(* Logix 5000 AddOnInstructionDefinition export POINT_ENC; software revision 30.00; part 2 of 2 *)

ADD_ON_INSTRUCTION B256_CtoE   (* revision 1.0 20170916, vendor Kenneth A. Fischer *)
// Convert 256-bit value using 22 12-bit pieces into 256-bit value using 32 8-bit pieces
// Revision note:
// Rev1.0: 20170916 - Initial Release
VAR_IN_OUT
   Inp_C : DINT[22]; {required}
   Out_E : DINT[32]; {required}
END_VAR
VAR
   i : INT;
   j : INT;
   TEMP1 : DINT;
   TEMP2 : DINT;
   D_SHL : D_SHL;
   D_SHR : D_SHR;
END_VAR

ROUTINE Logic   (* ladder *)
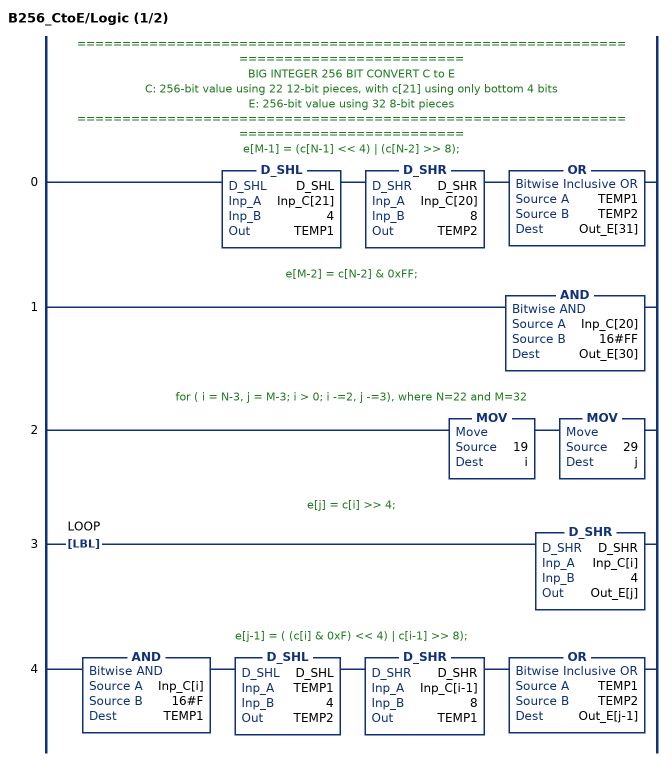
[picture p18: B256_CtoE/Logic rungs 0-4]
   // ======================================================================================
   // BIG INTEGER 256 BIT CONVERT C to E
   // C: 256-bit value using 22 12-bit pieces, with c[21] using only bottom 4 bits
   // E: 256-bit value using 32 8-bit pieces
   // ======================================================================================
   // e[M-1] = (c[N-1] << 4) | (c[N-2] >> 8);
   0: D_SHL(D_SHL,Inp_C[21],4,TEMP1)D_SHR(D_SHR,Inp_C[20],8,TEMP2)OR(TEMP1,TEMP2,Out_E[31]);
   // e[M-2] = c[N-2] & 0xFF;
   1: AND(Inp_C[20],16#FF,Out_E[30]);
   // for ( i = N-3, j = M-3; i > 0; i -=2, j -=3), where N=22 and M=32
   2: MOV(19,i)MOV(29,j);
   // e[j] = c[i] >> 4;
   3: LBL(LOOP)D_SHR(D_SHR,Inp_C[i],4,Out_E[j]);
   // e[j-1] = ( (c[i] & 0xF) << 4) | c[i-1] >> 8);
   4: AND(Inp_C[i],16#F,TEMP1)D_SHL(D_SHL,TEMP1,4,TEMP2)D_SHR(D_SHR,Inp_C[i-1],8,TEMP1)OR(TEMP1,TEMP2,Out_E[j-1]);
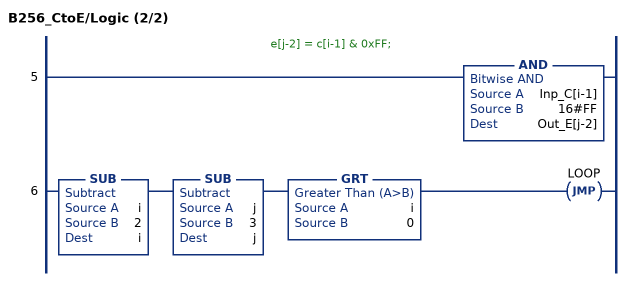
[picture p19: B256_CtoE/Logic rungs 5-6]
   // e[j-2] = c[i-1] & 0xFF;
   5: AND(Inp_C[i-1],16#FF,Out_E[j-2]);
   6: SUB(i,2,i)SUB(j,3,j)GRT(i,0)JMP(LOOP);
END_ROUTINE
END_ADD_ON_INSTRUCTION

ADD_ON_INSTRUCTION POINT_ENC   (* revision 1.0 20170916, vendor Kenneth A. Fischer *)
// Point Encode:
// Encode point (x,y) values into 32 8-bit pieces
// Requires POINT UDT
// Revision note:
// Rev1.0: 20170916 - Initial Release
VAR_IN_OUT
   Temp_C1 : DINT[22]; {required}
   Temp_C2 : DINT[22]; {required}
   Temp_C3 : DINT[22]; {required}
   Temp_C4 : DINT[22]; {required}   // U
   Temp_D : DINT[43]; {required}
   Temp_E : DINT[32]; {required}
   Inp_P : POINT; {required}
   Out_E : DINT[32]; {required}
END_VAR
VAR_OUTPUT
   i : INT; {access Read Only}
END_VAR
VAR_INPUT
   SEQCTRL_RESET : BOOL;   // Resets Point Multiplication if Toggled True
END_VAR
VAR_OUTPUT
   SEQCTRL_DN : BOOL; {access Read Only}   // Complete
   SEQCTRL_STEP : INT; {access Read Only}
END_VAR
VAR
   SEQCTRL_CMD : INT;
   SEQCTRL_DONE : INT;
   SEQCTRL_CMD_TABLE : INT[40];
   SEQCTRL_NEXT_STEP : INT;
   TEMP : INT;
   j : INT;
   b : DINT;
   B256_MUL : B256_MUL;
   B256_SQU : B256_SQU;
   B256_ADJ : B256_ADJ;
   B256_CtoE : B256_CtoE;
   D_SHL : D_SHL;
   TEMP1 : DINT;
   TEMP2 : DINT;
END_VAR

ROUTINE Logic   (* ladder *)
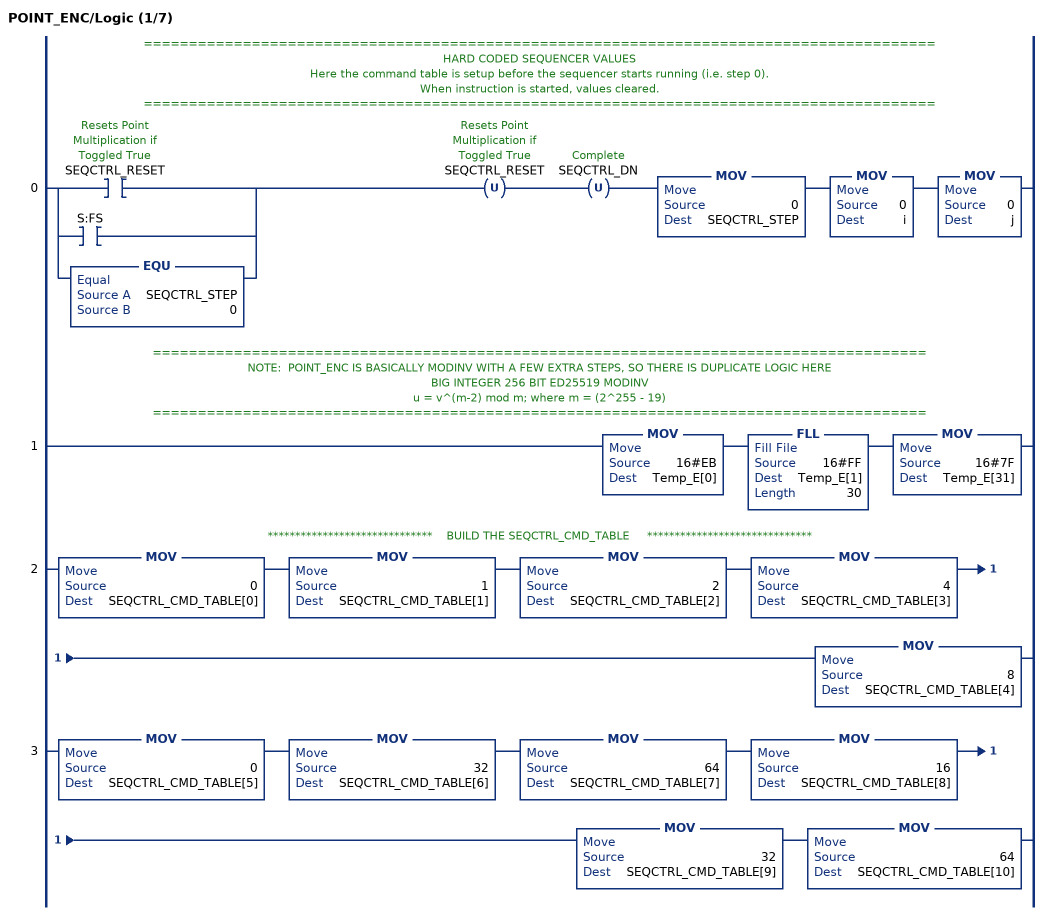
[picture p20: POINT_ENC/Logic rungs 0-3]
   // ========================================================================================
   // HARD CODED SEQUENCER VALUES
   // Here the command table is setup before the sequencer starts running (i.e. step 0).
   // When instruction is started, values cleared.
   // ========================================================================================
   0: [[XIC(SEQCTRL_RESET) ,XIC(S:FS) ] ,EQU(SEQCTRL_STEP,0) ]OTU(SEQCTRL_RESET)OTU(SEQCTRL_DN)MOV(0,SEQCTRL_STEP)MOV(0,i)MOV(0,j);
   // ======================================================================================
   // NOTE:  POINT_ENC IS BASICALLY MODINV WITH A FEW EXTRA STEPS, SO THERE IS DUPLICATE LOGIC HERE
   // BIG INTEGER 256 BIT ED25519 MODINV
   //  u = v^(m-2) mod m; where m = (2^255 - 19)
   // ======================================================================================
   1: MOV(16#EB,Temp_E[0])FLL(16#FF,Temp_E[1],30)MOV(16#7F,Temp_E[31]);
   // ******************************    BUILD THE SEQCTRL_CMD_TABLE     ******************************
   2: MOV(0,SEQCTRL_CMD_TABLE[0])MOV(1,SEQCTRL_CMD_TABLE[1])MOV(2,SEQCTRL_CMD_TABLE[2])MOV(4,SEQCTRL_CMD_TABLE[3])MOV(8,SEQCTRL_CMD_TABLE[4]);
   3: MOV(0,SEQCTRL_CMD_TABLE[5])MOV(32,SEQCTRL_CMD_TABLE[6])MOV(64,SEQCTRL_CMD_TABLE[7])MOV(16,SEQCTRL_CMD_TABLE[8])MOV(32,SEQCTRL_CMD_TABLE[9])MOV(64,SEQCTRL_CMD_TABLE[10]);
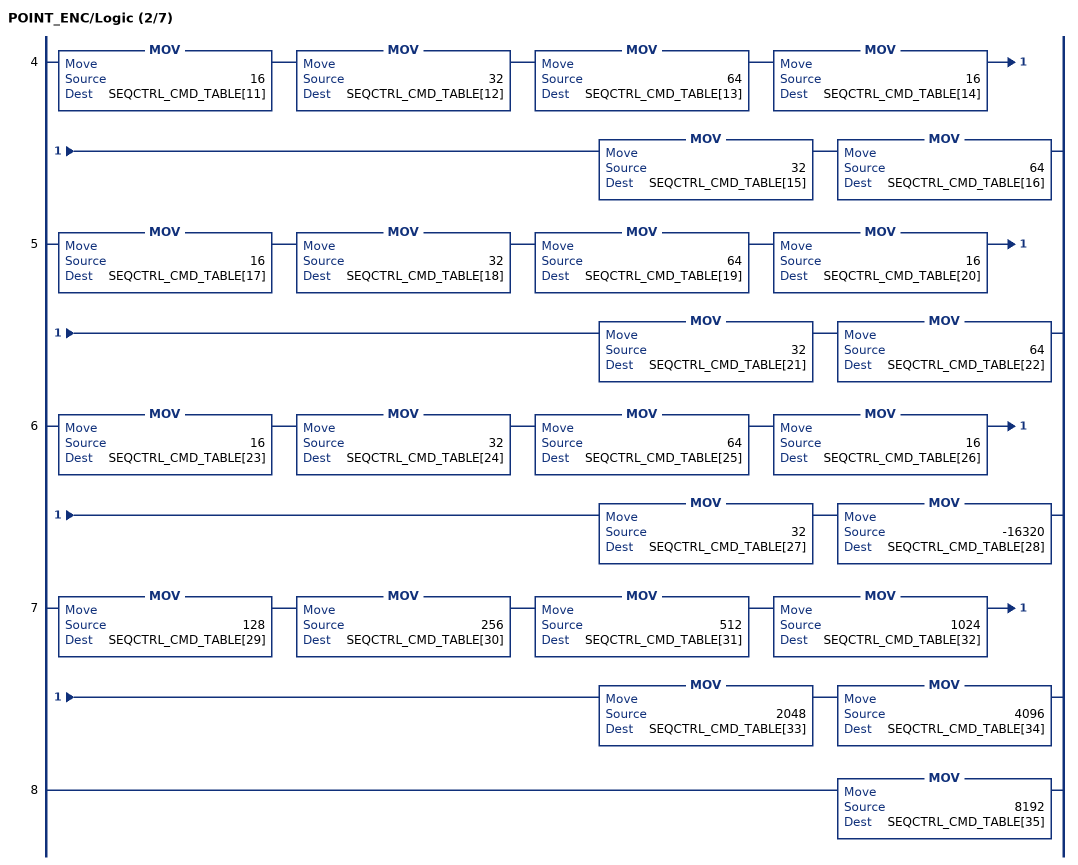
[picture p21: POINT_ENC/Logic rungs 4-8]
   4: MOV(16,SEQCTRL_CMD_TABLE[11])MOV(32,SEQCTRL_CMD_TABLE[12])MOV(64,SEQCTRL_CMD_TABLE[13])MOV(16,SEQCTRL_CMD_TABLE[14])MOV(32,SEQCTRL_CMD_TABLE[15])MOV(64,SEQCTRL_CMD_TABLE[16]);
   5: MOV(16,SEQCTRL_CMD_TABLE[17])MOV(32,SEQCTRL_CMD_TABLE[18])MOV(64,SEQCTRL_CMD_TABLE[19])MOV(16,SEQCTRL_CMD_TABLE[20])MOV(32,SEQCTRL_CMD_TABLE[21])MOV(64,SEQCTRL_CMD_TABLE[22]);
   6: MOV(16,SEQCTRL_CMD_TABLE[23])MOV(32,SEQCTRL_CMD_TABLE[24])MOV(64,SEQCTRL_CMD_TABLE[25])MOV(16,SEQCTRL_CMD_TABLE[26])MOV(32,SEQCTRL_CMD_TABLE[27])MOV(-16320,SEQCTRL_CMD_TABLE[28]);
   7: MOV(128,SEQCTRL_CMD_TABLE[29])MOV(256,SEQCTRL_CMD_TABLE[30])MOV(512,SEQCTRL_CMD_TABLE[31])MOV(1024,SEQCTRL_CMD_TABLE[32])MOV(2048,SEQCTRL_CMD_TABLE[33])MOV(4096,SEQCTRL_CMD_TABLE[34]);
   8: MOV(8192,SEQCTRL_CMD_TABLE[35]);
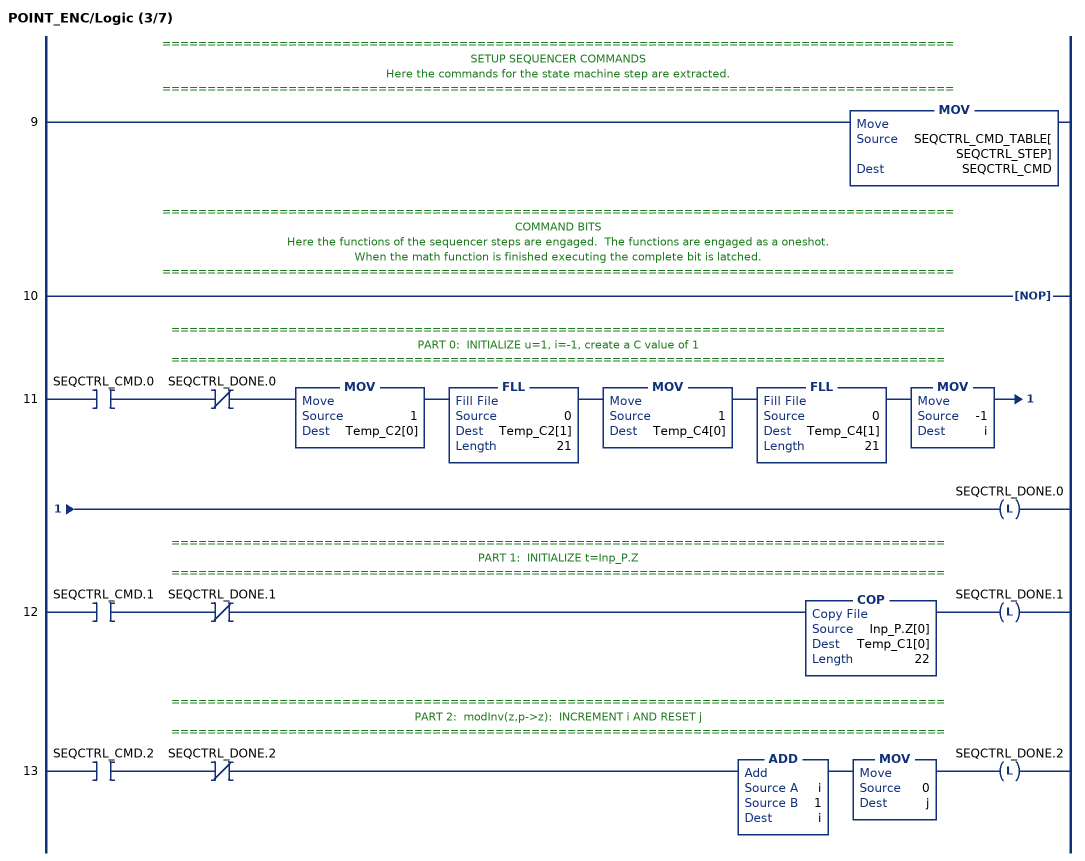
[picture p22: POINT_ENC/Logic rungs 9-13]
   // ========================================================================================
   // SETUP SEQUENCER COMMANDS
   // Here the commands for the state machine step are extracted.
   // ========================================================================================
   9: MOV(SEQCTRL_CMD_TABLE[SEQCTRL_STEP],SEQCTRL_CMD);
   // ========================================================================================
   // COMMAND BITS
   // Here the functions of the sequencer steps are engaged.  The functions are engaged as a oneshot.
   // When the math function is finished executing the complete bit is latched.
   // ========================================================================================
   10: NOP();
   // ======================================================================================
   // PART 0:  INITIALIZE u=1, i=-1, create a C value of 1
   // ======================================================================================
   11: XIC(SEQCTRL_CMD.0)XIO(SEQCTRL_DONE.0)MOV(1,Temp_C2[0])FLL(0,Temp_C2[1],21)MOV(1,Temp_C4[0])FLL(0,Temp_C4[1],21)MOV(-1,i)OTL(SEQCTRL_DONE.0);
   // ======================================================================================
   // PART 1:  INITIALIZE t=Inp_P.Z
   // ======================================================================================
   12: XIC(SEQCTRL_CMD.1)XIO(SEQCTRL_DONE.1)COP(Inp_P.Z[0],Temp_C1[0],22)OTL(SEQCTRL_DONE.1);
   // ======================================================================================
   // PART 2:  modInv(z,p->z):  INCREMENT i AND RESET j
   // ======================================================================================
   13: XIC(SEQCTRL_CMD.2)XIO(SEQCTRL_DONE.2)ADD(i,1,i)MOV(0,j)OTL(SEQCTRL_DONE.2);
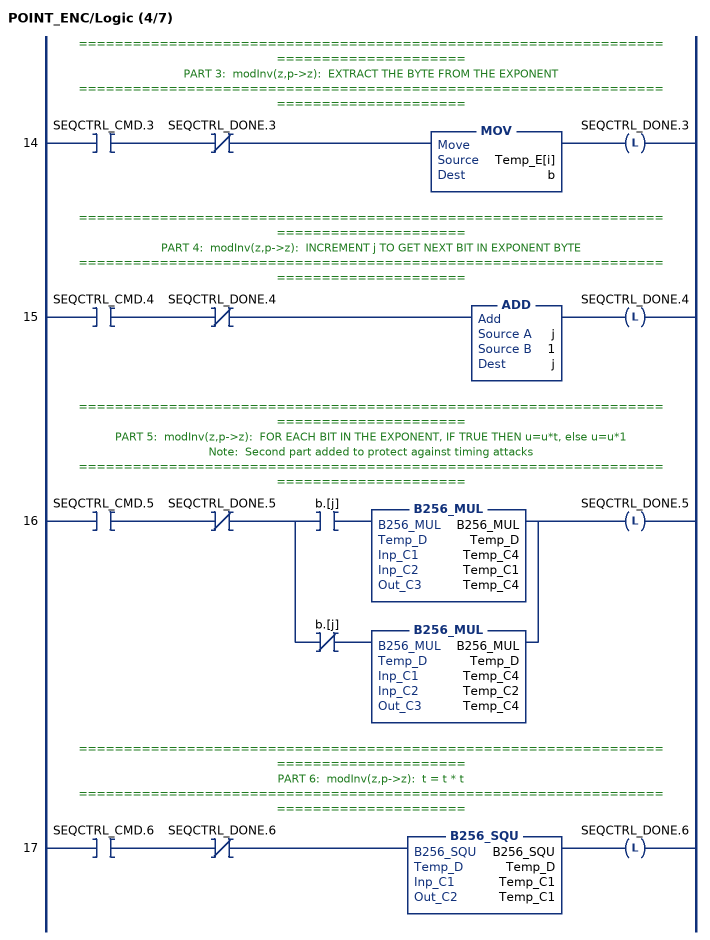
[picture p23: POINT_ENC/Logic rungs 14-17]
   // ======================================================================================
   // PART 3:  modInv(z,p->z):  EXTRACT THE BYTE FROM THE EXPONENT
   // ======================================================================================
   14: XIC(SEQCTRL_CMD.3)XIO(SEQCTRL_DONE.3)MOV(Temp_E[i],b)OTL(SEQCTRL_DONE.3);
   // ======================================================================================
   // PART 4:  modInv(z,p->z):  INCREMENT j TO GET NEXT BIT IN EXPONENT BYTE
   // ======================================================================================
   15: XIC(SEQCTRL_CMD.4)XIO(SEQCTRL_DONE.4)ADD(j,1,j)OTL(SEQCTRL_DONE.4);
   // ======================================================================================
   // PART 5:  modInv(z,p->z):  FOR EACH BIT IN THE EXPONENT, IF TRUE THEN u=u*t, else u=u*1
   // Note:  Second part added to protect against timing attacks
   // ======================================================================================
   16: XIC(SEQCTRL_CMD.5)XIO(SEQCTRL_DONE.5)[XIC(b.[j]) B256_MUL(B256_MUL,Temp_D,Temp_C4,Temp_C1,Temp_C4) ,XIO(b.[j]) B256_MUL(B256_MUL,Temp_D,Temp_C4,Temp_C2,Temp_C4) ]OTL(SEQCTRL_DONE.5);
   // ======================================================================================
   // PART 6:  modInv(z,p->z):  t = t * t
   // ======================================================================================
   17: XIC(SEQCTRL_CMD.6)XIO(SEQCTRL_DONE.6)B256_SQU(B256_SQU,Temp_D,Temp_C1,Temp_C1)OTL(SEQCTRL_DONE.6);
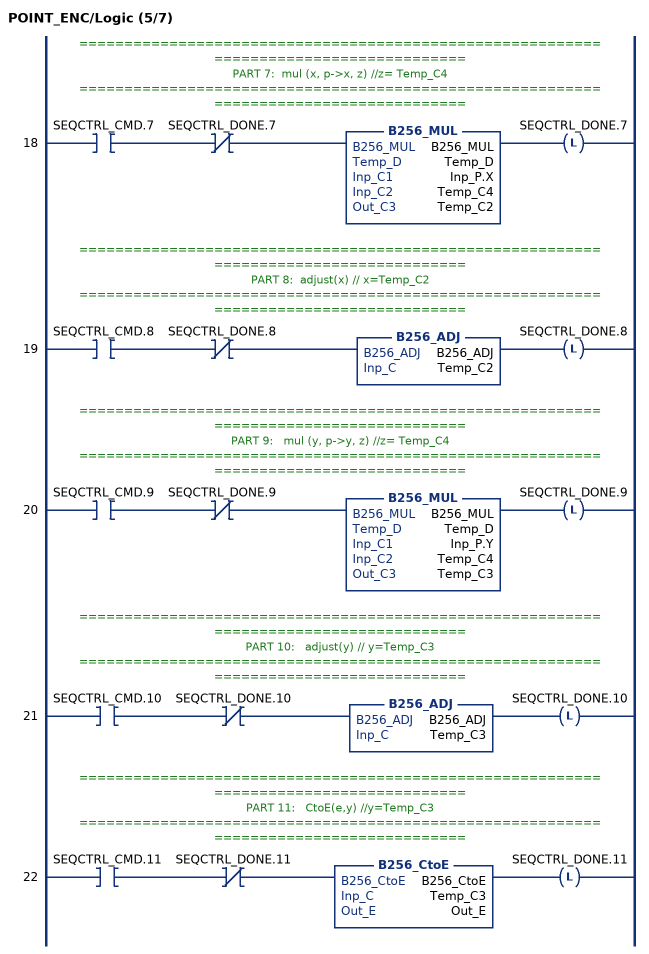
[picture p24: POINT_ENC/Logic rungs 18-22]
   // ======================================================================================
   // PART 7:  mul (x, p->x, z) //z= Temp_C4
   // ======================================================================================
   18: XIC(SEQCTRL_CMD.7)XIO(SEQCTRL_DONE.7)B256_MUL(B256_MUL,Temp_D,Inp_P.X,Temp_C4,Temp_C2)OTL(SEQCTRL_DONE.7);
   // ======================================================================================
   // PART 8:  adjust(x) // x=Temp_C2
   // ======================================================================================
   19: XIC(SEQCTRL_CMD.8)XIO(SEQCTRL_DONE.8)B256_ADJ(B256_ADJ,Temp_C2)OTL(SEQCTRL_DONE.8);
   // ======================================================================================
   // PART 9:   mul (y, p->y, z) //z= Temp_C4
   // ======================================================================================
   20: XIC(SEQCTRL_CMD.9)XIO(SEQCTRL_DONE.9)B256_MUL(B256_MUL,Temp_D,Inp_P.Y,Temp_C4,Temp_C3)OTL(SEQCTRL_DONE.9);
   // ======================================================================================
   // PART 10:   adjust(y) // y=Temp_C3
   // ======================================================================================
   21: XIC(SEQCTRL_CMD.10)XIO(SEQCTRL_DONE.10)B256_ADJ(B256_ADJ,Temp_C3)OTL(SEQCTRL_DONE.10);
   // ======================================================================================
   // PART 11:   CtoE(e,y) //y=Temp_C3
   // ======================================================================================
   22: XIC(SEQCTRL_CMD.11)XIO(SEQCTRL_DONE.11)B256_CtoE(B256_CtoE,Temp_C3,Out_E)OTL(SEQCTRL_DONE.11);
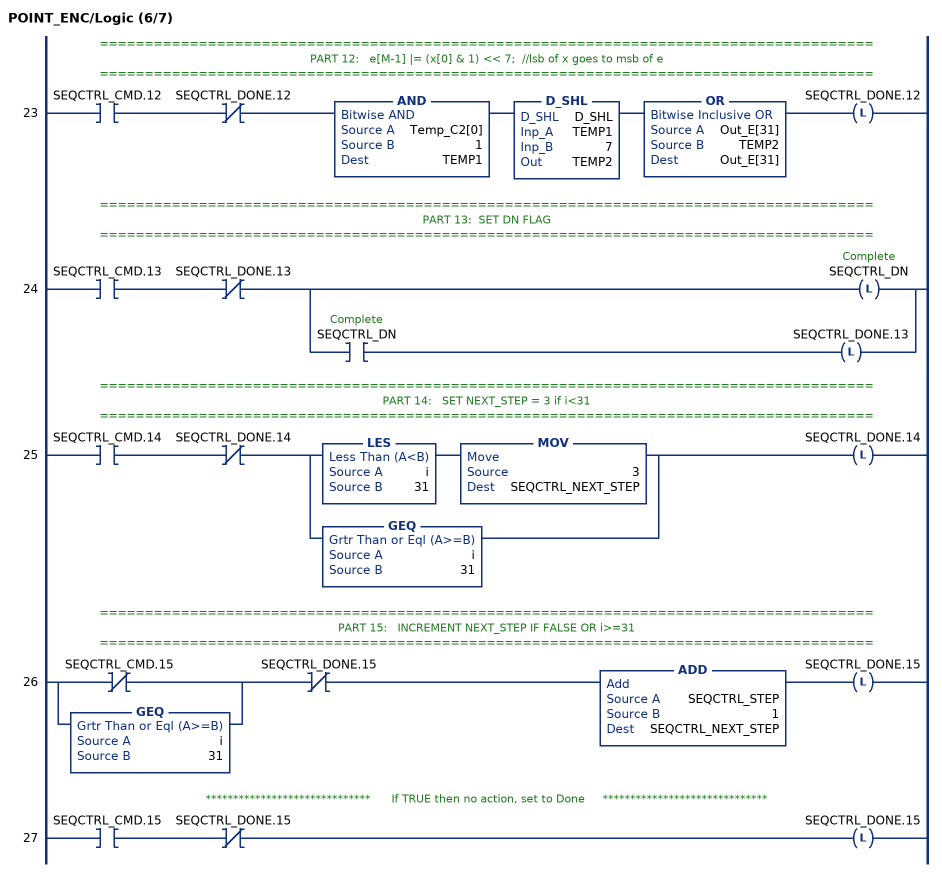
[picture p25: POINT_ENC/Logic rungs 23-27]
   // ======================================================================================
   // PART 12:   e[M-1] |= (x[0] & 1) << 7;  //lsb of x goes to msb of e
   // ======================================================================================
   23: XIC(SEQCTRL_CMD.12)XIO(SEQCTRL_DONE.12)AND(Temp_C2[0],1,TEMP1)D_SHL(D_SHL,TEMP1,7,TEMP2)OR(Out_E[31],TEMP2,Out_E[31])OTL(SEQCTRL_DONE.12);
   // ======================================================================================
   // PART 13:  SET DN FLAG
   // ======================================================================================
   24: XIC(SEQCTRL_CMD.13)XIO(SEQCTRL_DONE.13)[OTL(SEQCTRL_DN) ,XIC(SEQCTRL_DN) OTL(SEQCTRL_DONE.13) ];
   // ======================================================================================
   // PART 14:   SET NEXT_STEP = 3 if i<31
   // ======================================================================================
   25: XIC(SEQCTRL_CMD.14)XIO(SEQCTRL_DONE.14)[LES(i,31) MOV(3,SEQCTRL_NEXT_STEP) ,GEQ(i,31) ]OTL(SEQCTRL_DONE.14);
   // ======================================================================================
   // PART 15:   INCREMENT NEXT_STEP IF FALSE OR i>=31
   // ======================================================================================
   26: [XIO(SEQCTRL_CMD.15) ,GEQ(i,31) ]XIO(SEQCTRL_DONE.15)ADD(SEQCTRL_STEP,1,SEQCTRL_NEXT_STEP)OTL(SEQCTRL_DONE.15);
   // ******************************      If TRUE then no action, set to Done     ******************************
   27: XIC(SEQCTRL_CMD.15)XIO(SEQCTRL_DONE.15)OTL(SEQCTRL_DONE.15);
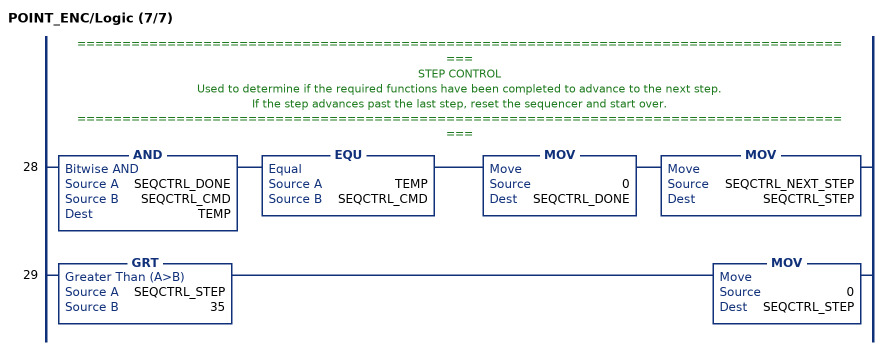
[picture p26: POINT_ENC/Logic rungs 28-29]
   // ========================================================================================
   // STEP CONTROL
   // Used to determine if the required functions have been completed to advance to the next step.
   // If the step advances past the last step, reset the sequencer and start over.
   // ========================================================================================
   28: AND(SEQCTRL_DONE,SEQCTRL_CMD,TEMP)EQU(TEMP,SEQCTRL_CMD)MOV(0,SEQCTRL_DONE)MOV(SEQCTRL_NEXT_STEP,SEQCTRL_STEP);
   29: GRT(SEQCTRL_STEP,35)MOV(0,SEQCTRL_STEP);
END_ROUTINE
END_ADD_ON_INSTRUCTION
